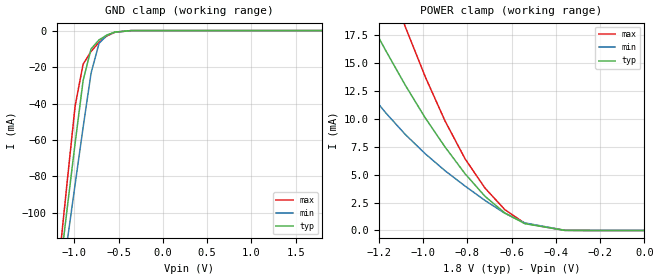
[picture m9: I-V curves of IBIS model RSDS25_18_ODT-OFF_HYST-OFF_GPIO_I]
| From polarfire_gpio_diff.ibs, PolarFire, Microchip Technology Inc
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|   Model RSDS25_18_ODT-OFF_HYST-OFF_GPIO_I
[Model]   RSDS25_18_ODT-OFF_HYST-OFF_GPIO_I
Model_type   Input
Vinl =   1.125
Vinh =   1.375
|   typ   min   max
C_comp_pullup   2.605e-12   2.605e-12   2.76e-12
C_comp_pulldown  2.605e-12   2.605e-12   2.76e-12
[Temperature Range]  25C   100C   -40C
[Voltage Range]  1.8   1.71   1.89
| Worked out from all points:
|   GND clamp passes 1 mA (typ) near -0.55 V on its own axis
|   POWER clamp passes 1 mA (typ) near -0.58 V on its own axis
[GND_clamp]
|Voltage   I(typ)   I(min)   I(max)
-1.8V     -400.9mA   -379.8mA   -437.5mA
-1.17V    -134.2mA   -147.8mA   -125.8mA
-1.08V    -97.7mA    -115.9mA   -83.09mA
-990mV    -61.78mA   -84.35mA   -41.33mA
-900mV    -27.45mA   -53.17mA   -18.47mA
-810mV    -10.06mA   -23.34mA   -11.43mA
-720mV    -5.122mA   -7.016mA   -6.424mA
-630mV    -2.387mA   -2.536mA   -2.907mA
-540mV    -812.6uA   -895.6uA   -914.9uA
-360mV    -11.27uA   -22.35uA   -9.971uA
1.8V      703.8nA    823.4nA    606.9nA
[POWER_clamp]
|Voltage   I(typ)   I(min)   I(max)
-1.8V     43.47mA    30.55mA    65.7mA
-1.44V    26.56mA    17.78mA    40.91mA
-1.26V    19.47mA    12.78mA    28.82mA
-1.17V    16.17mA    10.57mA    23.39mA
-1.08V    13.01mA    8.597mA    18.22mA
-900mV    7.463mA    5.343mA    9.787mA
-810mV    5.079mA    3.976mA    6.415mA
-720mV    3.058mA    2.687mA    3.796mA
-630mV    1.563mA    1.536mA    1.86mA
-540mV    609.2uA    674.8uA    644.4uA
-360mV    10.61uA    19.82uA    9.534uA
0V        0A         0A         0A
